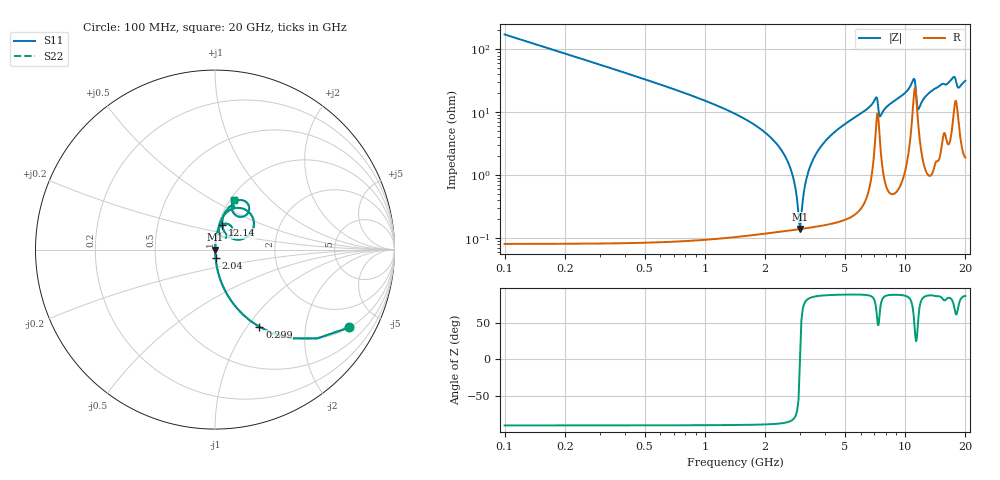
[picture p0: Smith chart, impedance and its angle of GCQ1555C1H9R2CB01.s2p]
!Murata Part Number: GCQ1555C1H9R2CB01
!These Parameters are Measured in Series Mode Connection
!Data Generated on Mar 13, 2026
!  o--ll--o
!Port1  Port2
!  o------o
!Operation Temp=25[degC], DC Bias Voltage=0[V]
!Freq. Start=100[MHz] Stop=20[GHz] 401[Steps]
# Hz S RI R 50
!Freq.(Hz) S11(Real) S11(Imag) S21(Real) S21(Imag) S12(Real) S12(Imag) S22(Real) S22(Imag)
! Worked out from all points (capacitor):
!   401 points, 100 MHz to 20 GHz, reference 50 ohm
!   read as one part in series: C = 9.2 pF near 199.5 MHz
!   lowest |Z| = 140 mohm at 2.986 GHz (marker M1)
!   series resonance near 2.986 GHz, so ESL is about 310 pH
!   S11 on the Smith chart (normalised r, x): 100 MHz: 1.00, -3.46; 299 MHz: 1.00, -1.15; 2.04 GHz: 1.00, -0.09; 12.14 GHz: 1.04, +0.29; 20 GHz: 1.04, +0.64
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1e8  0.749 -0.4333  0.251 0.4333  0.251 0.4333  0.749 -0.4333
2.99e8  0.2473 -0.4307  0.7527 0.4307  0.7527 0.4307  0.2473 -0.4307
6.97e8  0.053 -0.2221  0.947 0.2221  0.947 0.2221  0.053 -0.2221
2.04025e9  0.00324 -0.0451  0.9968 0.0451  0.9968 0.0451  0.00324 -0.0451
2.63725e9  0.00153 -0.0145  0.9985 0.0145  0.9985 0.0145  0.00153 -0.0145
2.9855e9  0.0014 -1.14e-05  0.9986 1.14e-05  0.9986 1.14e-05  0.0014 -1.14e-05
3.085e9  0.00143 0.00381  0.9986 -0.00381  0.9986 -0.00381  0.00143 0.00381
3.23425e9  0.00154 0.00935  0.9985 -0.00935  0.9985 -0.00935  0.00154 0.00935
3.43325e9  0.00176 0.0164  0.9982 -0.0164  0.9982 -0.0164  0.00176 0.0164
4.42825e9  0.00404 0.0479  0.996 -0.0479  0.996 -0.0479  0.00404 0.0479
6.7665e9  0.0248 0.1252  0.9752 -0.1252  0.9752 -0.1252  0.0248 0.1252
7.1645e9  0.0782 0.1407  0.9218 -0.1407  0.9218 -0.1407  0.0782 0.1407
7.51275e9  0.0354 0.076  0.9646 -0.076  0.9646 -0.076  0.0354 0.076
1.005e10  0.0519 0.1939  0.9481 -0.1939  0.9481 -0.1939  0.0519 0.1939
1.099525e10  0.1836 0.2135  0.8164 -0.2135  0.8164 -0.2135  0.1836 0.2135
1.159225e10  0.0745 0.0739  0.9255 -0.0739  0.9255 -0.0739  0.0745 0.0739
1.21395e10  0.0401 0.1381  0.9599 -0.1381  0.9599 -0.1381  0.0401 0.1381
1.338325e10  0.0513 0.1986  0.9487 -0.1986  0.9487 -0.1986  0.0513 0.1986
1.67165e10  0.1127 0.2662  0.8873 -0.2662  0.8873 -0.2662  0.1127 0.2662
1.756225e10  0.181 0.2575  0.819 -0.2575  0.819 -0.2575  0.181 0.2575
1.8408e10  0.1156 0.1913  0.8844 -0.1913  0.8844 -0.1913  0.1156 0.1913
2e10  0.1057 0.2787  0.8943 -0.2787  0.8943 -0.2787  0.1057 0.2787
